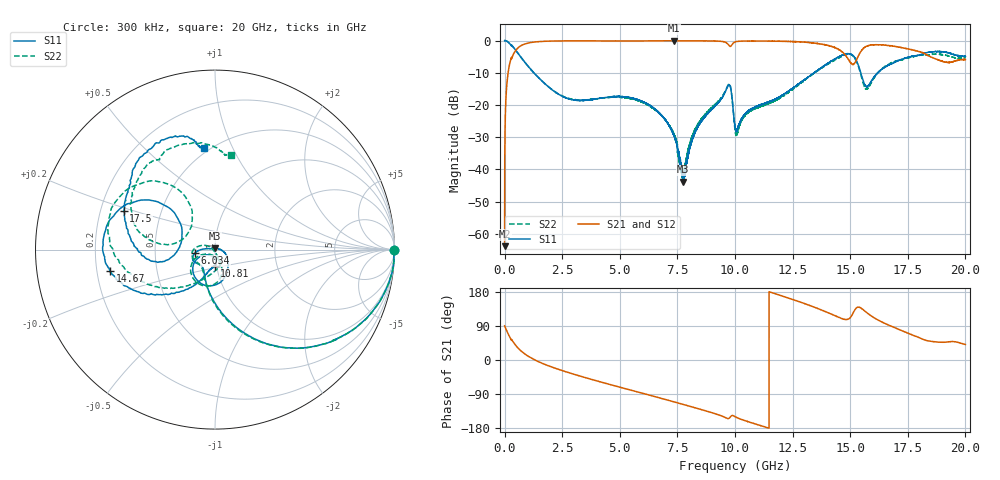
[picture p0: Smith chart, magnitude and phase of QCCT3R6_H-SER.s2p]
!{QCCT3R6}
!Johanson Technology Inc.
!www.johansontechnology.com
!Test Board Conditions:
!Substrate Type  RO4350B
!Substrate Thickness  20 mil
!Substrate Dk  3.66
!TL Type: GCPW
!TL Trace Width  34 mil
!TL Gap  10 mil
!Electrode orientation  Horizontal
!DUT TOPOLOGY	SERIES
!Mounting Pad LxW  26x52 mil
# MHz S  dB  R 50
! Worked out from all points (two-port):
!   20001 points, 300 kHz to 20 GHz, reference 50 ohm
!   highest |S21| = -0.05 dB at 7.367 GHz (marker M1); lowest = -63.8 dB at 300 kHz (marker M2)
!   |S21| within 3 dB of the highest: 484 MHz to 14.57 GHz (14.09 GHz wide, 187 % of centre); 15.5 GHz to 17.79 GHz (2.294 GHz wide, 13.8 % of centre)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
!   lowest |S11| = -43.8 dB at 7.757 GHz (marker M3), VSWR 1.01, Z = 50.1 + j0.642 ohm
!   |S11| at or under -10 dB: 1.27 GHz to 13.43 GHz (12.16 GHz wide, 165 % of centre); 15.46 GHz to 16.2 GHz (737.7 MHz wide, 4.66 % of centre); 16.19669 GHz to 16.19862 GHz (1.922 MHz wide, 0.0119 % of centre)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
!   |S22| runs from -43.0 to 0.0 dB; largest |S21 - S12| = 0.021
!   S11 on the Smith chart (normalised r, x): 300 kHz: open; 6.034 GHz: 0.80, -0.03; 10.81 GHz: 0.98, -0.18; 14.67 GHz: 0.26, -0.09; 17.5 GHz: 0.30, +0.18; 20 GHz: 0.47, +0.78
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0.3  -0.03 -0.1  -63.79 90.3  -64.15 87.0  -0.02 -0.3
119.298  -0.29 -16.4  -11.93 73.3  -11.90 73.3  -0.29 -16.4
378.294  -2.07 -42.5  -4.31 47.1  -4.29 47.1  -2.08 -42.6
1280.281  -10.09 -88.4  -0.47 1.2  -0.48 1.1  -10.09 -89.2
3334.25  -18.60 -131.2  -0.10 -43.5  -0.10 -43.5  -18.47 -135.1
6034.209  -19.08 -171.0  -0.11 -88.5  -0.11 -88.5  -19.33 174.3
6667.2  -22.14 -179.9  -0.09 -99.0  -0.10 -99.0  -22.24 162.5
7367.189  -29.91 169.7  -0.05 -110.7  -0.07 -110.8  -29.36 151.3
7757.184  -43.77 81.6  -0.06 -117.3  -0.07 -117.3  -41.34 -128.9
8330.175  -27.48 -8.4  -0.09 -127.3  -0.09 -127.1  -27.03 -68.4
9697.155  -14.06 -90.6  -1.13 -154.6  -1.12 -154.4  -13.79 -98.3
9823.153  -15.12 -134.3  -1.74 -148.4  -1.72 -148.4  -14.96 -139.5
10000.15  -26.60 -139.5  -0.45 -149.5  -0.44 -149.4  -27.71 -142.8
10810.14  -20.84 -91.7  -0.14 -167.4  -0.14 -167.3  -21.36 -70.2
13334.1  -10.51 -129.1  -0.69 141.9  -0.65 141.8  -10.65 -133.7
14670.08  -4.49 -168.4  -3.62 108.9  -3.60 108.7  -4.74 178.5
15203.07  -5.43 151.1  -6.91 132.2  -7.01 132.1  -5.51 133.8
15711.06  -14.32 165.2  -1.75 125.4  -1.78 125.1  -15.03 148.4
16667.05  -7.65 -177.5  -1.53 92.1  -1.72 92.1  -7.34 167.3
17504.04  -5.16 157.3  -2.61 70.8  -2.61 70.8  -5.42 150.5
18859.02  -3.40 113.8  -6.09 47.0  -6.06 46.8  -4.26 105.8
20000  -4.91 96.3  -5.91 40.9  -5.99 41.2  -5.43 80.6
